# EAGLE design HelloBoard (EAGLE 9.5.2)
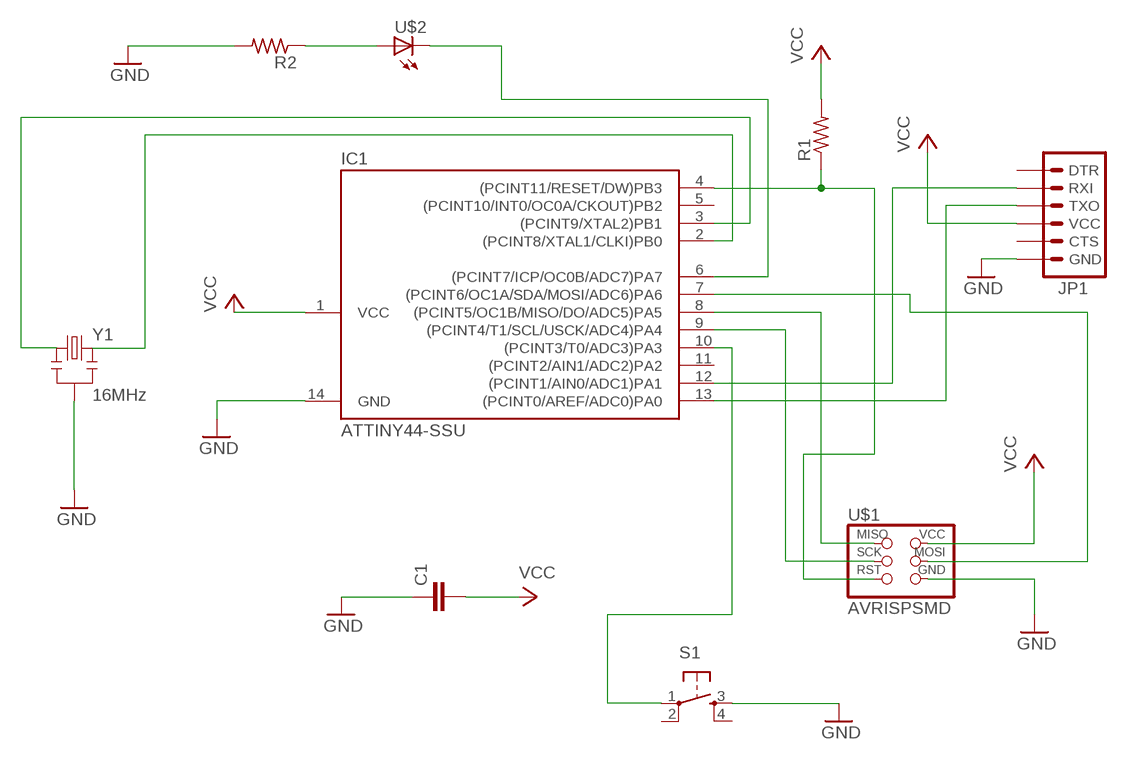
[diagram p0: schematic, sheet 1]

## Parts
C1  C-EUC1206  [C1206]
IC1  ATTINY44-SSU  [SOIC14]
JP1  FTDI_CONNECTORSMD  [1X06]
R1  RESISTOR1206  [1206]
R2  RESISTOR1206  [1206]
S1  6MM_SWITCH6MM_SWITCH  [6MM_SWITCH]
U$1  AVRISPSMD  [2X03SMD]
U$2  LED1206  [1206]
Y1  16MHz  RESONATOR16MHZ  [RESONATOR-SMD]

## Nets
GND: C1.1 IC1.14(GND) JP1.6(GND) R2.2 S1.3(S) U$1.6(GND) Y1.2
N$1: R2.1 U$2.1(A)
N$2: IC1.6((PCINT7/ICP/OC0B/ADC7)PA7) U$2.2(C)
N$3: IC1.4((PCINT11/RESET/DW)PB3) R1.1 U$1.5(RST)
N$4: IC1.12((PCINT1/AIN0/ADC1)PA1) JP1.2(RXI)
N$5: IC1.2((PCINT8/XTAL1/CLKI)PB0) Y1.3
N$6: IC1.3((PCINT9/XTAL2)PB1) Y1.1
N$7: IC1.10((PCINT3/T0/ADC3)PA3) S1.1(P)
N$8: IC1.9((PCINT4/T1/SCL/USCK/ADC4)PA4) U$1.3(SCK)
N$9: IC1.8((PCINT5/OC1B/MISO/DO/ADC5)PA5) U$1.1(MISO)
N$10: IC1.13((PCINT0/AREF/ADC0)PA0) JP1.3(TXO)
N$12: IC1.7((PCINT6/OC1A/SDA/MOSI/ADC6)PA6) U$1.4(MOSI)
VCC: C1.2 IC1.1(VCC) JP1.4(VCC) R1.2 U$1.2(VCC)
Unconnected: IC1.5((PCINT10/INT0/OC0A/CKOUT)PB2) IC1.11((PCINT2/AIN1/ADC2)PA2) JP1.1(DTR) JP1.5(CTS) S1.2(P1) S1.4(S1)

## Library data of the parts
C1 = rcl:C-EU: CAPACITOR, European symbol; SPICEPREFIX: C
IC1 = fablab:ATTINY44
JP1 = fablab:FTDI_CONNECTOR: FTDI connector smd
R1 R2 = fablab:RESISTOR
S1 = fablab:6MM_SWITCH: OMRON SWITCH
U$1 = fablab:AVRISP
U$2 = fablab:LED
Y1 = fablab:RESONATOR: Resonator Small SMD resonator. Used, eg, on the Arduino Pro/ Pro Mini boards. 8MHz- XTAL-08895 16MHz- XTAL-08900; PROD_ID: XTAL-08900

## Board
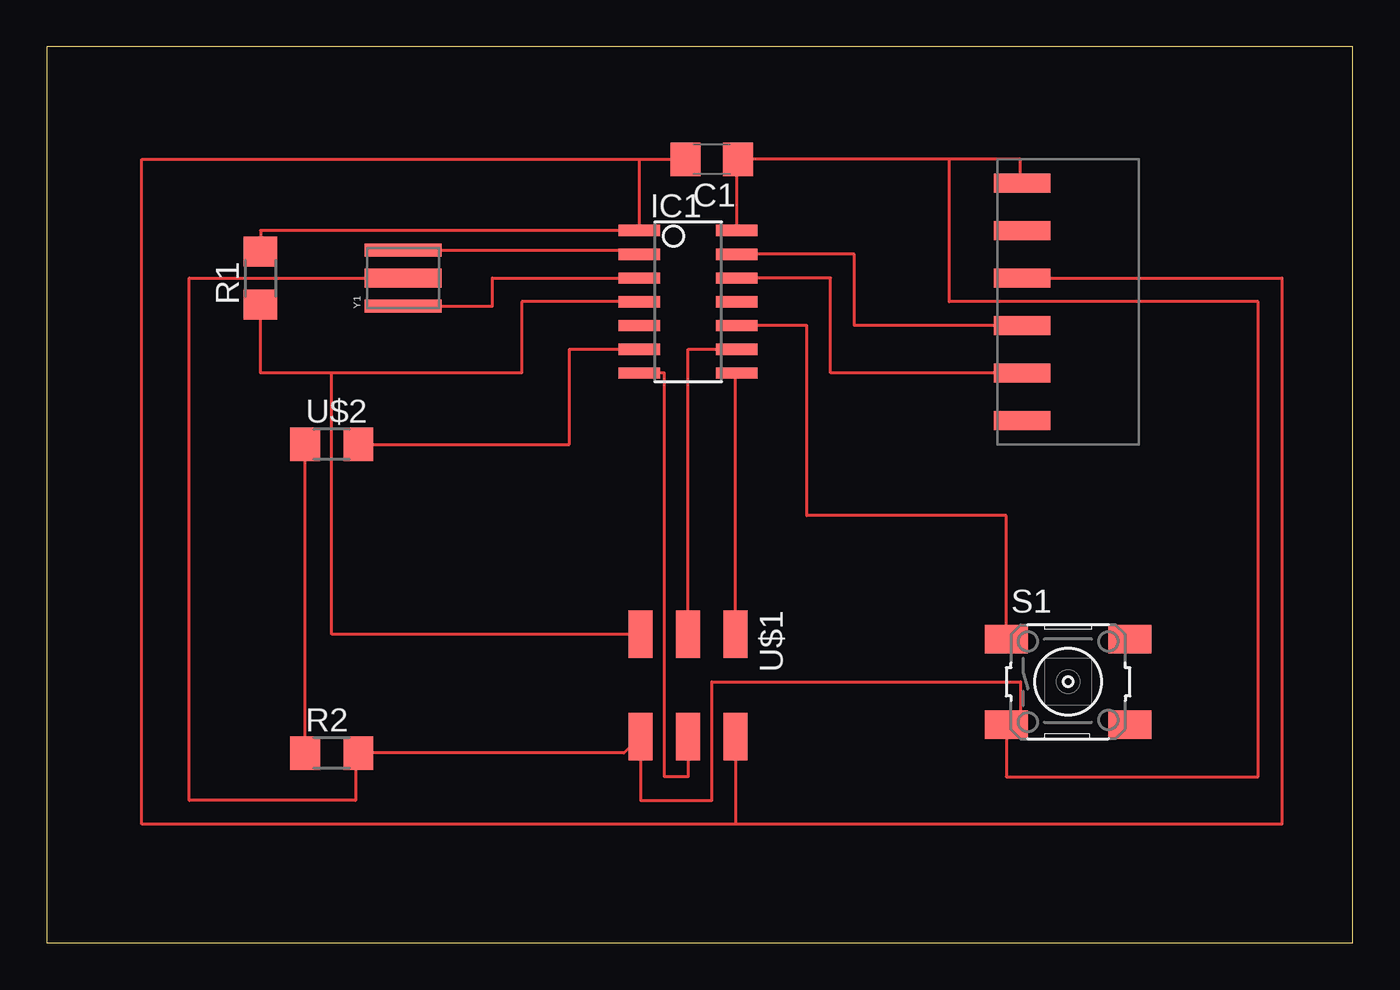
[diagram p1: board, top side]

Size 69.83 x 47.93 mm. Coordinates in mm from the lower left corner, seen from the top.
Outline: 0,0 69.83,0 69.83,47.93 0,47.93 0,0
Copper layers (1*16): Top 0.035mm / dielectric 1.5mm / Bottom 0.035mm
Design rules "default *": minimum track width 6mil, minimum drill 0.35mm, track to track 6mil, track to pad 6mil, pad to pad 6mil, via to via 6mil, smd to smd 6mil, copper to edge 40mil, drill to drill 6mil, minimum pad ring 10mil, minimum via ring 8mil, stop-mask expansion 4mil, vias tented up to drill 0mil, thermal gap 10mil

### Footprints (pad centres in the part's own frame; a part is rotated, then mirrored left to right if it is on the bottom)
C1206 = smd 1.6 x 1.8: 1 -1.4,0; 2 1.4,0
SOIC14 = smd 0.61 x 2.21: 1 -3.81,-2.603; 2 -2.54,-2.603; 3 -1.27,-2.603; 4 0,-2.603; 5 1.27,-2.603; 6 2.54,-2.603; 7 3.81,-2.603; 8 3.81,2.603; 9 2.54,2.603; 10 1.27,2.603; 11 0,2.603; 12 -1.27,2.603; 13 -2.54,2.603; 14 -3.81,2.603
1X06 = smd 1 x 3: 1 -6.35,5; 2 -3.81,5; 3 -1.27,5; 4 1.27,5; 5 3.81,5; 6 6.35,5
1206 = smd 1.6 x 1.803: 1 -1.422,0; 2 1.422,0
6MM_SWITCH = smd 2.286 x 1.524: 1 -3.302,2.286; 2 3.302,2.286; 3 -3.302,-2.286; 4 3.302,-2.286
2X03SMD = smd 2.54 x 1.27: 1 -2.54,2.54; 2 2.92,2.54; 3 -2.54,0; 4 2.92,0; 5 -2.54,-2.54; 6 2.92,-2.54
RESONATOR-SMD = smd 0.7 x 4.1: 1 -1.5,0; 3 1.5,0 | smd 1 x 4.1: 2 0,0

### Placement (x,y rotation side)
C1  35.56,41.91 180 top
IC1  34.29,34.29 270 top
JP1  57.15,34.29 90 top
R1  11.43,35.56 90 top
R2  15.24,10.16 0 top
S1  54.61,13.97 0 top
U$1  34.29,13.97 270 top
U$2  15.24,26.67 0 top
Y1  19.05,35.56 90 top

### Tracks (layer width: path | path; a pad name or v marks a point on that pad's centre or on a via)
GND
  Top 0.152: 53.34,40.64 JP1.6 52.07,40.64 52.07,41.91 48.26,41.91 | 48.26,41.91 C1.1 36.89,41.91 IC1.14 | 20.32,35.56 Y1.2 7.62,35.56 7.62,7.62 16.51,7.62 16.51,10.16 R2.2 30.86,10.16 U$1.6 31.75,7.62 35.56,7.62 35.56,13.97 52.07,13.97 52.07,11.43 51.31,11.43 | S1.3 51.31,11.43 | 51.31,11.43 51.31,8.89 64.77,8.89 64.77,34.29 48.26,34.29 48.26,41.91
N$1
  Top 0.152: R2.1 U$2.1
N$2
  Top 0.152: U$2.2 27.94,26.67 27.94,31.75 IC1.6
N$3
  Top 0.152: 15.24,30.48 25.4,30.48 25.4,34.29 IC1.4 | 15.24,30.48 11.43,30.48 R1.1 | U$1.5 15.24,16.51 15.24,30.48
N$4
  Top 0.152: IC1.12 41.91,35.56 41.91,30.48 JP1.2
N$5
  Top 0.152: Y1.3 31.69,37.06 IC1.2
N$6
  Top 0.152: 19.05,34.29 Y1.1 23.82,34.06 23.82,34.29 23.82,34.82 23.82,35.56 IC1.3 31.75,35.56
N$7
  Top 0.152: S1.1 51.31,22.86 40.64,22.86 40.64,33.02 IC1.10
N$8
  Top 0.152: U$1.3 34.29,31.75 IC1.9
N$9
  Top 0.152: U$1.1 36.83,30.48 IC1.8
N$10
  Top 0.152: IC1.13 43.18,36.83 43.18,33.02 JP1.3
N$12
  Top 0.152: U$1.4 34.29,8.89 33.02,8.89 33.02,30.48 IC1.7
VCC
  Top 0.152: JP1.4 66.04,35.56 66.04,6.35 36.83,6.35 | U$1.2 36.83,6.35 | C1.2 5.08,41.91 5.08,6.35 36.83,6.35 | R1.2 11.43,38.1 IC1.1 31.69,41.91 C1.2 | 34.29,41.91 C1.2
